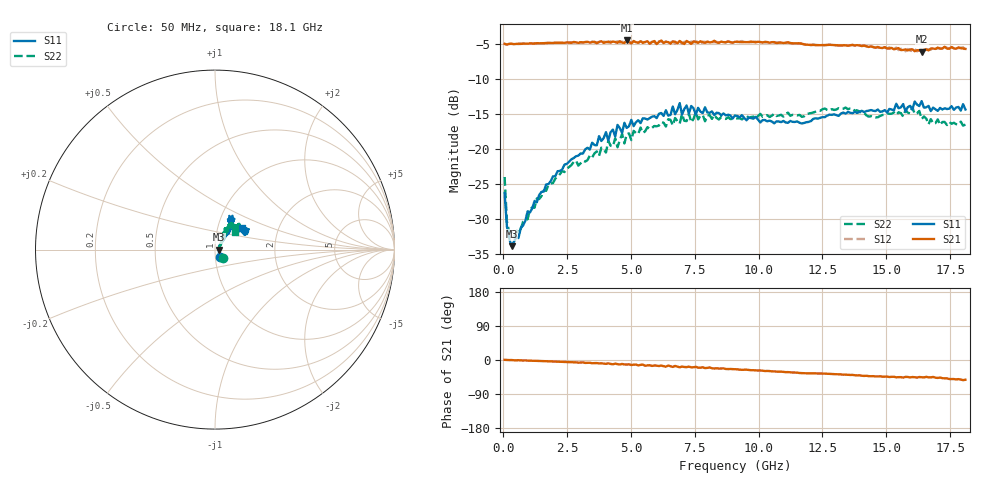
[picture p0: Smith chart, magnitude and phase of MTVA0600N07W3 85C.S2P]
! Network Analyzer HP8720D.06.14 Serial No. US36140669
!  8 Jul 2005  12:41:10
! Frequency  S11  S21  S12  S22
# HZ  S  DB R 50
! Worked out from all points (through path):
!   201 points, 50 MHz to 18.1 GHz, reference 50 ohm
!   highest |S21| = -4.52 dB at 4.833 GHz (marker M1); lowest = -6.1 dB at 16.39 GHz (marker M2)
!   group delay of S21, straight-line fit = 8.32 ps
!   lowest |S11| = -33.9 dB at 320.8 MHz (marker M3), VSWR 1.04, Z = 52.1 - j0.111 ohm
!   |S11| at or under -10 dB: start of sweep to end of sweep
!   |S22| runs from -32.6 to -14.0 dB; largest |S21 - S12| = 0.029
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5e7  -26.29 -58.4  -4.99 0.4  -5.03 0.7  -24.02 -47.1
1.4025e8  -31.09 -36.9  -5.10 0.0  -5.08 -0.0  -30.39 -32.7
3.2075e8  -33.90 -3.0  -4.98 -0.1  -5.01 -0.1  -31.99 -4.6
1.6745e9  -25.09 45.8  -4.90 -3.2  -4.88 -3.2  -25.99 49.1
3.1185e9  -20.67 52.9  -4.79 -6.4  -4.83 -6.8  -21.68 58.4
4.021e9  -17.61 55.3  -4.76 -10.2  -4.75 -9.1  -20.52 58.3
4.11125e9  -18.82 55.6  -4.69 -8.9  -4.81 -10.2  -18.84 58.6
4.47225e9  -16.58 51.9  -4.86 -10.9  -4.64 -10.2  -19.78 64.2
4.83325e9  -17.01 61.1  -4.52 -12.0  -4.77 -12.5  -17.89 55.0
6.09675e9  -14.99 57.7  -4.73 -16.0  -4.63 -15.9  -16.66 59.1
6.7285e9  -15.06 65.2  -4.71 -15.6  -4.98 -16.3  -15.59 55.1
6.909e9  -13.46 62.8  -4.59 -19.3  -4.66 -17.5  -16.40 54.7
6.99925e9  -15.09 62.8  -4.82 -17.2  -5.01 -19.1  -15.03 56.2
7.17975e9  -13.80 67.0  -4.59 -18.8  -4.83 -17.4  -16.04 51.7
7.54075e9  -15.12 59.5  -4.73 -18.0  -4.65 -20.8  -14.73 59.3
9.075e9  -15.23 61.0  -4.71 -24.4  -4.69 -24.5  -15.63 49.9
1.21435e10  -15.71 45.3  -5.15 -35.1  -5.09 -35.3  -14.81 48.1
1.512175e10  -14.29 28.0  -5.68 -44.9  -5.50 -44.7  -15.00 46.8
1.602425e10  -14.38 32.2  -5.79 -45.0  -6.03 -47.1  -14.05 41.3
1.638525e10  -13.18 31.1  -6.13 -45.4  -5.89 -44.8  -15.74 39.7
1.674625e10  -14.60 33.4  -5.66 -45.9  -5.84 -46.5  -15.75 42.3
1.81e10  -14.38 38.0  -5.72 -52.1  -5.87 -52.6  -16.53 41.1
